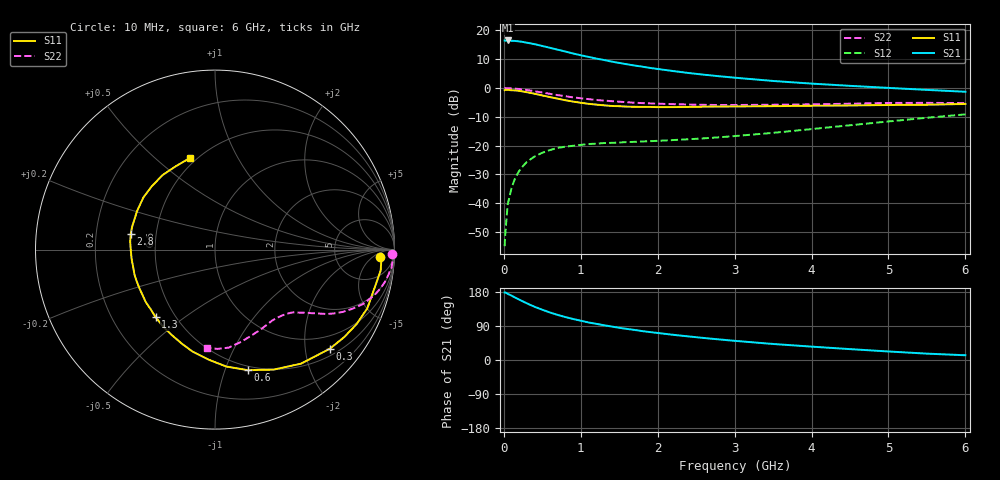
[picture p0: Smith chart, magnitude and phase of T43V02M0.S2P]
! Infineon Technologies  Discrete & RF Semiconductors
! BFR182T
! Si NPN RF Bipolar Junction Transistor in SC75
! VCE = 3 V  IC = 2 mA
! Common Emitter S-Parameters:  October  1999
# GHz  S  MA  R  50
!  f  S11  S21  S12  S22
! GHz  MAG  ANG  MAG  ANG  MAG  ANG  MAG  ANG
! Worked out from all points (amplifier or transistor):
!   36 points, 10 MHz to 6 GHz, reference 50 ohm
!   highest |S21| = 16.5 dB at 50 MHz (marker M1)
!   |S21| within 3 dB of that: start of sweep to 668 MHz
!   unconditionally stable (mu >= 1): 1.98 GHz to 4.342 GHz
!   at 250 MHz: K = 0.14, MSG = 21.5 dB, |S12| = -27.1 dB
!   at 1.4 GHz: K = 0.78, MSG = 14.1 dB, |S12| = -19.0 dB
!   at 6 GHz: K = 0.82, MSG = 3.9 dB, |S12| = -9.1 dB
!   lowest NFmin = 1.10 dB at 450 MHz
!   S11 on the Smith chart (normalised r, x): 10 MHz: 19, -10; 300 MHz: 0.66, -2.55; 600 MHz: 0.46, -1.20; 1.3 GHz: 0.39, -0.39; 2.8 GHz: 0.36, +0.08; 6 GHz: 0.46, +0.65
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0.01  0.9185 -2.5  6.668 178.3  0.0018 78.4  0.9892 -1.4
0.02  0.9295 -1.4  6.656 178.3  0.0031 85.3  0.9971 -1.1
0.05  0.9304 -7.2  6.699 174.7  0.0095 87.9  0.9929 -2.9
0.1  0.9141 -13.6  6.608 169.9  0.0184 82.5  0.9885 -5.8
0.15  0.9095 -21.1  6.562 164.4  0.0281 78.2  0.9751 -8.5
0.2  0.8915 -27.7  6.449 159.3  0.0365 75.9  0.9616 -11.1
0.3  0.8457 -40.7  6.123 149.5  0.0526 68.1  0.9245 -15.9
0.4  0.7959 -53.0  5.776 140.4  0.0649 61.8  0.8796 -20.1
0.5  0.744 -64.0  5.375 132.6  0.0753 57.0  0.8351 -23.2
0.6  0.6962 -74.8  4.988 125.3  0.0839 53.1  0.7938 -25.9
0.8  0.6137 -93.4  4.303 113.3  0.096 46.8  0.72 -29.9
0.9  0.582 -102.4  3.982 108.2  0.0994 45.2  0.6888 -31.2
1.1  0.532 -117.5  3.476 99.1  0.1066 42.1  0.6416 -33.5
1.3  0.5013 -131.3  3.07 91.8  0.1109 40.8  0.6048 -35.5
1.5  0.4839 -142.9  2.731 85.0  0.1134 40.6  0.5798 -37.2
1.8  0.4706 -158.3  2.35 76.2  0.1182 41.4  0.5476 -40.1
2.2  0.4675 -173.4  1.974 66.5  0.1251 44.0  0.5256 -44.1
2.8  0.4778 169.2  1.603 54.3  0.1397 49.5  0.5074 -51.5
3.5  0.4846 153.5  1.327 42.3  0.1668 55.3  0.5129 -60.4
4.5  0.4983 135.2  1.092 28.7  0.2259 58.8  0.535 -74.7
5.5  0.5134 115.1  0.929 16.8  0.3049 56.9  0.5533 -88.6
6  0.529 105.4  0.862 12.5  0.3493 54.0  0.5482 -94.9
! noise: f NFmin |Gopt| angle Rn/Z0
0.45  1.1  0.42  29  0.36
0.9  1.2  0.4  58  0.3
1.8  1.85  0.32  126  0.22
